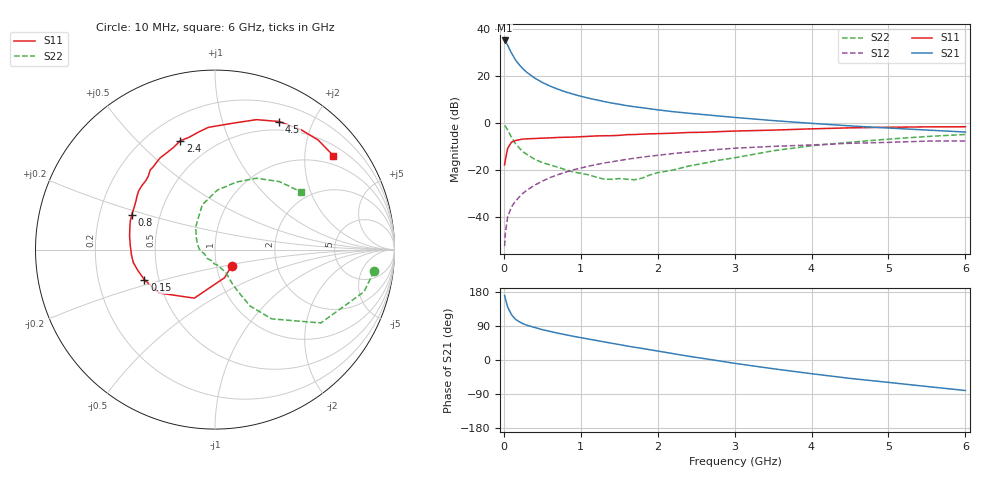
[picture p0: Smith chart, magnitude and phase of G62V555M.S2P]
! SIEMENS Small Signal Semiconductors
! BFG193
! Si NPN RF Bipolar Junction Transistor in SOT223
! VCE = 2.5 V  IC = 55 mA
! Common Emitter S-Parameters:  August  1996
# GHz  S  MA  R  50
!  f  S11  S21  S12  S22
! GHz  MAG  ANG  MAG  ANG  MAG  ANG  MAG  ANG
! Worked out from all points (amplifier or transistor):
!   36 points, 10 MHz to 6 GHz, reference 50 ohm
!   highest |S21| = 35.3 dB at 10 MHz (marker M1)
!   |S21| within 3 dB of that: start of sweep to 63.71 MHz
!   unconditionally stable (mu >= 1): 360.3 MHz to 2.384 GHz
!   at 250 MHz: K = 0.94, MSG = 26.5 dB, |S12| = -29.8 dB
!   at 1.4 GHz: K = 1.06, MAG = 11.0 dB, |S12| = -16.5 dB
!   at 6 GHz: K = 0.92, MSG = 1.9 dB, |S12| = -7.5 dB
!   S11 on the Smith chart (normalised r, x): 10 MHz: 1.18, -0.22; 150 MHz: 0.41, -0.17; 800 MHz: 0.34, +0.18; 2.4 GHz: 0.33, +0.68; 4.5 GHz: 0.39, +1.55; 6 GHz: 0.75, +2.68
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0.01  0.1296 -44.7  58.19 170.2  0.0024 82.4  0.8941 -7.8
0.02  0.1655 -71.3  55.61 161.7  0.0046 75.2  0.8629 -15.8
0.05  0.2941 -113.1  45.74 139.5  0.0101 70.2  0.7178 -34.7
0.1  0.3944 -142.2  31.23 119.5  0.0166 66.3  0.4989 -50.7
0.15  0.4277 -156.9  22.59 107.6  0.0217 66.6  0.3705 -58.1
0.2  0.4454 -164.9  17.7 101.0  0.0268 67.7  0.2985 -60.1
0.25  0.4608 -170.9  14.36 95.8  0.0324 68.1  0.2456 -61.9
0.3  0.4661 -176.0  12.13 91.8  0.0374 69.5  0.2161 -63.0
0.4  0.4728 177.0  9.216 85.9  0.0477 69.2  0.1713 -64.0
0.5  0.4818 171.0  7.4 80.1  0.0583 68.4  0.1451 -64.4
0.6  0.4884 166.4  6.206 75.5  0.0694 67.4  0.1298 -66.6
0.7  0.4977 161.6  5.343 70.9  0.0798 66.1  0.116 -70.3
0.8  0.5032 157.2  4.672 66.7  0.0903 63.8  0.1026 -73.9
1.1  0.5262 145.7  3.428 55.3  0.1214 58.5  0.0797 -91.9
1.3  0.5414 138.9  2.911 47.9  0.1419 54.3  0.0644 -108.8
1.6  0.5716 129.2  2.372 36.9  0.1705 47.2  0.0642 -142.1
2.2  0.6137 112.3  1.765 16.8  0.226 33.4  0.1007 164.1
2.4  0.6363 107.7  1.638 10.0  0.2425 29.1  0.122 148.3
3.5  0.7141 81.2  1.14 -23.0  0.322 1.5  0.259 106.0
4.5  0.7981 63.4  0.879 -48.5  0.3743 -18.5  0.3937 72.6
5.5  0.8385 46.7  0.716 -69.9  0.4164 -41.8  0.5222 46.5
6  0.8415 38.5  0.65 -80.5  0.4201 -55.1  0.5767 33.9
